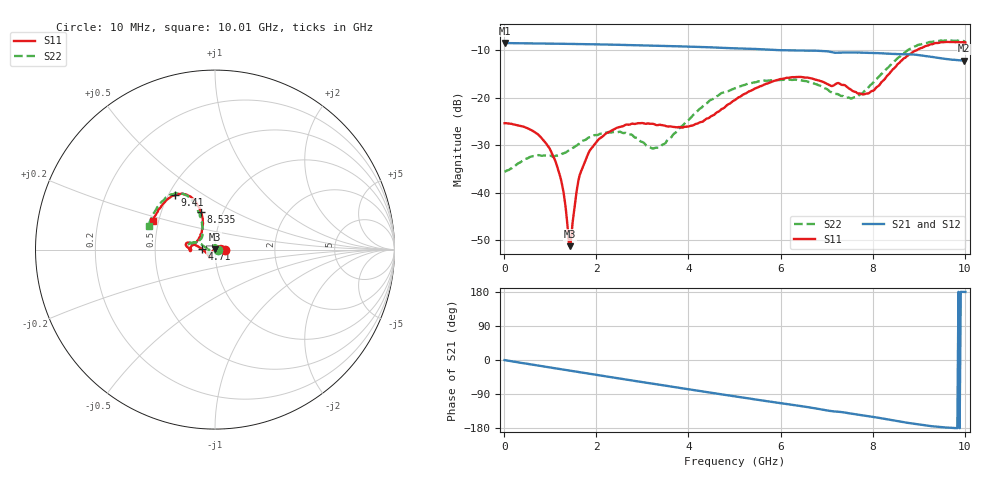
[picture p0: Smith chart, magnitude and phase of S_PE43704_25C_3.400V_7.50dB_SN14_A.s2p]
! Device ID: PE43704
! Dir: z:\PE43704\PE43704_Char_1_20130516\PE43704\AMB\3p400V\7p50dB
! Serial: 14
! Insertion: A
! Impedance: 50 ohm
! Temp: Amb
! VDD: 3.400V
! Attenuation Step: 7.50dB
! IDD: 1.140195e-01mA
#  Hz  S  RI  R  50
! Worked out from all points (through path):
!   401 points, 10 MHz to 10.01 GHz, reference 50 ohm
!   highest |S21| = -8.51 dB at 10 MHz (marker M1); lowest = -12.2 dB at 9.985 GHz (marker M2)
!   group delay of S21, straight-line fit = 51.5 ps
!   lowest |S11| = -51.3 dB at 1.435 GHz (marker M3), VSWR 1.01, Z = 49.8 + j0.144 ohm
!   |S11| at or under -10 dB: start of sweep to 8.957 GHz
!   |S22| runs from -35.6 to -8.0 dB; largest |S21 - S12| = 0.003
!   S11 on the Smith chart (normalised r, x): 10 MHz: 1.11, +0.00; 4.71 GHz: 0.86, +0.01; 8.535 GHz: 0.79, +0.35; 9.41 GHz: 0.54, +0.38; 10.01 GHz: 0.46, +0.17
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1e7  0.0538 0.00021  0.3755 -0.00145  0.3758 -0.00137  0.0165 0.000407
6.1e8  0.0408 0.0191  0.3639 -0.0785  0.3638 -0.0785  0.007 0.0231
9.85e8  0.0228 0.0183  0.3493 -0.1233  0.3493 -0.1232  -0.00761 0.0232
1.235e9  0.00881 0.0104  0.3363 -0.1522  0.3364 -0.1521  -0.0192 0.0164
1.385e9  -3.72e-05 0.00393  0.3272 -0.1686  0.3274 -0.1685  -0.0254 0.0102
1.435e9  -0.00231 0.00145  0.3241 -0.1738  0.3241 -0.1738  -0.0274 0.00791
1.585e9  -0.0103 -0.00462  0.314 -0.1897  0.3141 -0.1895  -0.0316 0.000924
1.685e9  -0.0141 -0.0103  0.3069 -0.2  0.307 -0.1998  -0.0345 -0.00364
2.235e9  -0.0277 -0.0322  0.2619 -0.2499  0.262 -0.2498  -0.0376 -0.021
3.36e9  -0.0321 -0.0407  0.1481 -0.3184  0.1485 -0.3182  -0.0289 -0.00711
4.035e9  -0.0455 -0.0214  0.0725 -0.3361  0.0729 -0.336  -0.0581 0.0156
4.71e9  -0.075 0.0044  -0.0035 -0.3346  -0.00317 -0.3345  -0.1035 0.0408
5.01e9  -0.093 0.0167  -0.0343 -0.3284  -0.0341 -0.3286  -0.1202 0.0366
5.96e9  -0.1497 0.0393  -0.1229 -0.2913  -0.122 -0.2915  -0.1493 0.0337
6.685e9  -0.158 0.017  -0.1847 -0.2515  -0.1848 -0.2513  -0.1389 0.0344
7.585e9  -0.1107 0.0357  -0.2368 -0.1826  -0.2367 -0.1824  -0.0746 0.0674
7.96e9  -0.0809 0.0834  -0.2545 -0.1505  -0.2544 -0.1511  -0.07 0.1178
8.36e9  -0.0685 0.1655  -0.2676 -0.1114  -0.267 -0.1125  -0.0851 0.1963
8.535e9  -0.0793 0.2094  -0.2721 -0.0928  -0.2716 -0.0948  -0.1048 0.2375
9.41e9  -0.2222 0.3029  -0.2623 -0.0171  -0.262 -0.0163  -0.2601 0.296
9.985e9  -0.3417 0.1673  -0.2452 0.00181  -0.2462 0.00281  -0.3649 0.1421
1.001e10  -0.3474 0.1569  -0.2456 0.00202  -0.2473 0.00225  -0.3689 0.1337
